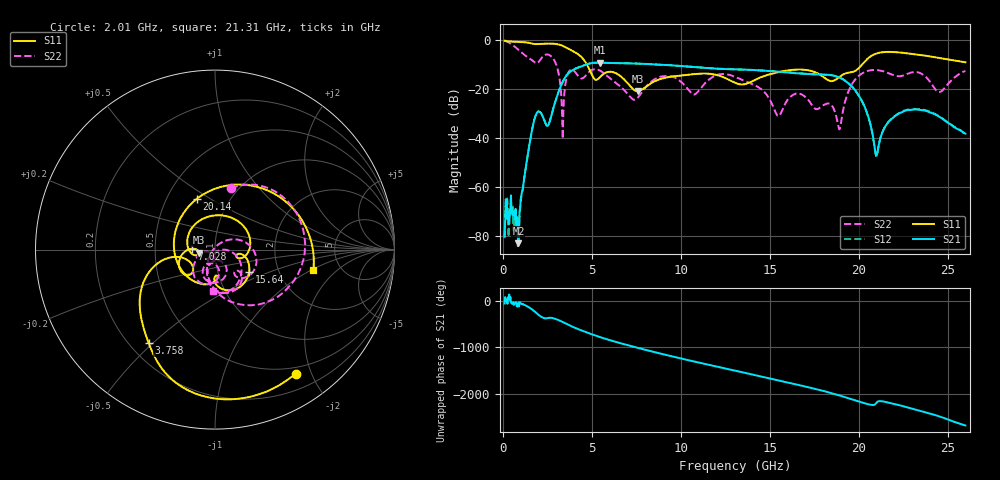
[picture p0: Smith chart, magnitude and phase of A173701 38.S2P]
!  2-Port S-parameters saved by WinCal
! VAR MeasName=S-Parameters (CALIBRATED_DATA) read from VNA (N5245A)
! VAR MeasDate=2017-6-7 10:30:57
! VAR NAME=A173701 38
! VAR FILENAME=A173701 38.S2P
! VAR DATE=2017-6-7 10:30:57
! VAR PHYS_PORTS=1,2
# Hz S DB R 50
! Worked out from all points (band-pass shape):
!   801 points, 100 MHz to 26 GHz, reference 50 ohm
!   highest |S21| = -9.24 dB at 5.442 GHz (marker M1); lowest = -83.0 dB at 877 MHz (marker M2)
!   |S21| within 3 dB of the highest: 3.937 GHz to 14.09 GHz (10.16 GHz wide, 113 % of centre)
!   lowest |S11| = -20.9 dB at 7.611 GHz (marker M3), VSWR 1.20, Z = 41.9 - j1.5 ohm
!   |S11| at or under -10 dB: 4.723 GHz to 20.19 GHz (15.47 GHz wide, 124 % of centre)
!   |S22| runs from -40.4 to -0.2 dB; largest |S21 - S12| = 0.0044
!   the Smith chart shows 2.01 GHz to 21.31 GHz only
!   S11 on the Smith chart (normalised r, x): 2.01 GHz: 0.41, -1.77; 3.758 GHz: 0.28, -0.48; 7.028 GHz: 0.77, +0.01; 15.64 GHz: 1.41, -0.37; 20.14 GHz: 0.70, +0.44; 21.31 GHz: 3.18, -1.03
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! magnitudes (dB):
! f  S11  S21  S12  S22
! 100 MHz  -0.3  -80.0  -80.8  -0.2
! 877 MHz  -0.8  -83.0  -77.6  -4.0
! 1.589 GHz  -1.4  -38.8  -38.7  -8.0
! 2.01 GHz  -1.7  -29.1  -29.2  -9.0
! 2.884 GHz  -1.6  -26.7  -26.6  -8.2
! 3.37 GHz  -2.4  -17.0  -16.9  -40.4
! 3.758 GHz  -3.9  -13.1  -13.1  -12.5
! 4.438 GHz  -7.1  -10.7  -10.6  -15.7
! 5.442 GHz  -15.3  -9.2  -9.2  -12.4
! 7.028 GHz  -17.7  -9.5  -9.5  -22.2
! 7.611 GHz  -20.9  -9.7  -9.7  -23.3
! 8.744 GHz  -16.2  -10.1  -10.1  -15.3
! 13.05 GHz  -17.5  -12.0  -12.0  -15.1
! 15.64 GHz  -12.9  -13.0  -13.0  -29.7
! 17.39 GHz  -12.7  -14.0  -13.9  -26.7
! 18.91 GHz  -15.1  -15.4  -15.3  -36.5
! 20.14 GHz  -10.5  -24.2  -24.4  -13.9
! 20.98 GHz  -5.6  -47.3  -47.2  -12.3
! 21.31 GHz  -5.0  -38.2  -38.1  -12.6
! 21.69 GHz  -4.9  -33.3  -33.2  -13.6
! 24.54 GHz  -7.4  -31.4  -31.2  -21.2
! 26 GHz  -9.1  -38.2  -38.1  -12.6
